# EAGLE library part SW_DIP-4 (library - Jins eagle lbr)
DIP SWITCH
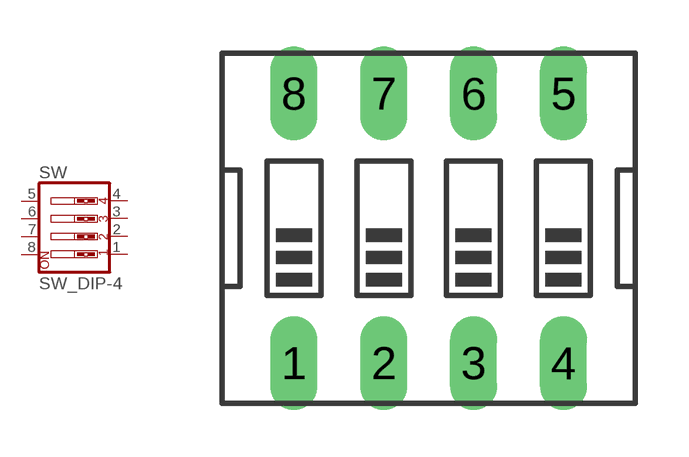
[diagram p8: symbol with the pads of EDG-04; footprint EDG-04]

Designator prefix SW

## SW_DIP-4  [EDG-04]
1  1  pas
2  2  pas
3  3  pas
4  4  pas
5  5  pas
6  6  pas
7  7  pas
8  8  pas

## Footprint EDG-04 (pad centres in mm)
DIP SWITCH
drill 0.813 long: 1 -3.81,-3.81; 2 -1.27,-3.81; 3 1.27,-3.81; 4 3.81,-3.81; 5 3.81,3.81; 6 1.27,3.81; 7 -1.27,3.81; 8 -3.81,3.81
